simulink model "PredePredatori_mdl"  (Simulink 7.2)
settings: Solver=ode45  StartTime=0.0  StopTime=10.0  RelTol=1e-3
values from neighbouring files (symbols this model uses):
  a = 0.9    [Exercises04a.m]
  b = 0.01    [Exercises04a.m]    (also in Exercises04b.m = 0.75)
  c = 0.8    [Exercises04a.m]
  d = 0.01    [Exercises04a.m]
  x0 = [70; 70]    [Exercises04a.m]    (also in Exercises04b.m = xe(2))

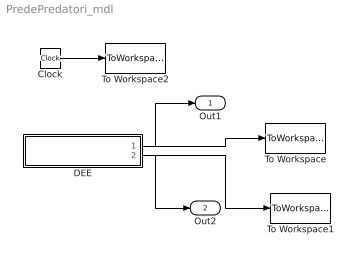
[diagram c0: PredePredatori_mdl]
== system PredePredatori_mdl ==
  Clock : Clock
  DEE : Subsystem
  To Workspace : ToWorkspace  VariableName=x1  SampleTime=-1  SaveFormat=Array
  To Workspace1 : ToWorkspace  VariableName=x2  SampleTime=-1  SaveFormat=Array
  To Workspace2 : ToWorkspace  VariableName=time  SampleTime=-1  SaveFormat=Array
  Out1 : Outport  OutDataType=sfix(16)  OutScaling=2^0
  Out2 : Outport  Port=2  OutDataType=sfix(16)  OutScaling=2^0
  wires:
  DEE/1(Port1) -> To Workspace/1, Out1/1
  DEE/2(Port2) -> To Workspace1/1, Out2/1
  Clock/1 -> To Workspace2/1

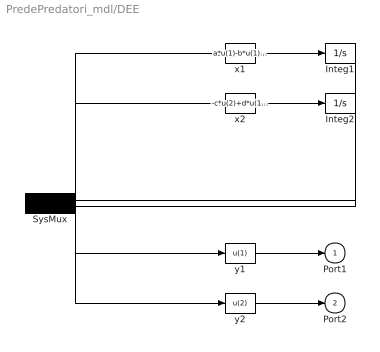
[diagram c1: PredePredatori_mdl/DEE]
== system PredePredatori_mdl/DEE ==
  Integ1 : Integrator  InitialCondition=x0(1)
  Integ2 : Integrator  InitialCondition=x0(2)
  SysMux : Mux  Inputs=2
  x1 : Fcn  Expr=a*u(1)-b*u(1)*u(2)
  x2 : Fcn  Expr=-c*u(2)+d*u(1)*u(2)
  y1 : Fcn  Expr=u(1)
  y2 : Fcn  Expr=u(2)
  Port1 : Outport
  Port2 : Outport  Port=2
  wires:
  SysMux/1 -> x1/1, x2/1, y1/1, y2/1
  x1/1 -> Integ1/1
  Integ1/1 -> SysMux/1
  x2/1 -> Integ2/1
  Integ2/1 -> SysMux/2
  y1/1 -> Port1/1
  y2/1 -> Port2/1
